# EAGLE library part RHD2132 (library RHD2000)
Intan Technologies RHD2132 chip
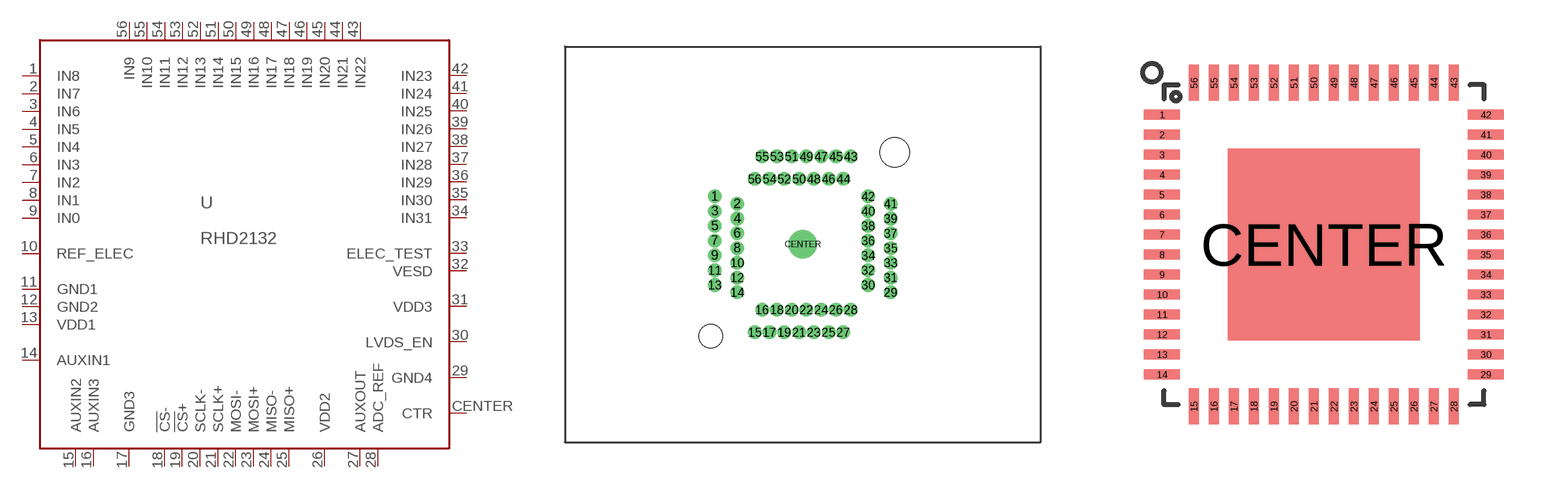
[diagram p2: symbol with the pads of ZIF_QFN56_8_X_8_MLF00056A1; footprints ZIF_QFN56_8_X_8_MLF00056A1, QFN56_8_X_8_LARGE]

Designator prefix U

## RHD2132_ZIF  [ZIF_QFN56_8_X_8_MLF00056A1]
1  IN8  in
2  IN7  in
3  IN6  in
4  IN5  in
5  IN4  in
6  IN3  in
7  IN2  in
8  IN1  in
9  IN0  in
10  REF_ELEC  in
11  GND1  pwr
12  GND2  pwr
13  VDD1  pwr
14  AUXIN1  in
15  AUXIN2  in
16  AUXIN3  in
17  GND3  pwr
18  !CS!-  in
19  !CS!+  in
20  SCLK-  in
21  SCLK+  in
22  MOSI-  in
23  MOSI+  in
24  MISO-  out
25  MISO+  out
26  VDD2  pwr
27  AUXOUT  hiz
28  ADC_REF  pas
29  GND4  pwr
30  LVDS_EN  in
31  VDD3  pwr
32  VESD  pwr
33  ELEC_TEST  in
34  IN31  in
35  IN30  in
36  IN29  in
37  IN28  in
38  IN27  in
39  IN26  in
40  IN25  in
41  IN24  in
42  IN23  in
43  IN22  in
44  IN21  in
45  IN20  in
46  IN19  in
47  IN18  in
48  IN17  in
49  IN16  in
50  IN15  in
51  IN14  in
52  IN13  in
53  IN12  in
54  IN11  in
55  IN10  in
56  IN9  in
CENTER  CTR  pwr

## RHD2132_QFN  [QFN56_8_X_8_LARGE]
Pads as for ZIF_QFN56_8_X_8_MLF00056A1

## RHD2132_COB  [RHD2000_56PIN_COB]
Pads as for ZIF_QFN56_8_X_8_MLF00056A1

## Footprint ZIF_QFN56_8_X_8_MLF00056A1 (pad centres in mm)
drill 0.41 pad 0.813: 1 -5.955,3.25; 2 -4.43,2.75; 3 -5.955,2.25; 4 -4.43,1.75; 5 -5.955,1.25; 6 -4.43,0.75; 7 -5.955,0.25; 8 -4.43,-0.25; 9 -5.955,-0.75; 10 -4.43,-1.25; 11 -5.955,-1.75; 12 -4.43,-2.25; 13 -5.955,-2.75; 14 -4.43,-3.25; 15 -3.25,-5.955; 16 -2.75,-4.43; 17 -2.25,-5.955; 18 -1.75,-4.43; 19 -1.25,-5.955; 20 -0.75,-4.43; 21 -0.25,-5.955; 22 0.25,-4.43; 23 0.75,-5.955; 24 1.25,-4.43; 25 1.75,-5.955; 26 2.25,-4.43; 27 2.75,-5.955; 28 3.25,-4.43; 29 5.955,-3.25; 30 4.43,-2.75; 31 5.955,-2.25; 32 4.43,-1.75; 33 5.955,-1.25; 34 4.43,-0.75; 35 5.955,-0.25; 36 4.43,0.25; 37 5.955,0.75; 38 4.43,1.25; 39 5.955,1.75; 40 4.43,2.25; 41 5.955,2.75; 42 4.43,3.25; 43 3.25,5.955; 44 2.75,4.43; 45 2.25,5.955; 46 1.75,4.43; 47 1.25,5.955; 48 0.75,4.43; 49 0.25,5.955; 50 -0.25,4.43; 51 -0.75,5.955; 52 -1.25,4.43; 53 -1.75,5.955; 54 -2.25,4.43; 55 -2.75,5.955; 56 -3.25,4.43
drill 1.2 pad 1.93: CENTER 0,0
hole 2 at 6.225,6.225
hole 1.6 at -6.225,-6.225

## Footprint QFN56_8_X_8_LARGE (pad centres in mm)
smd 0.9 x 0.25: 1 -4.05,3.25; 2 -4.05,2.75; 3 -4.05,2.25; 4 -4.05,1.75; 5 -4.05,1.25; 6 -4.05,0.75; 7 -4.05,0.25; 8 -4.05,-0.25; 9 -4.05,-0.75; 10 -4.05,-1.25; 11 -4.05,-1.75; 12 -4.05,-2.25; 13 -4.05,-2.75; 14 -4.05,-3.25; 29 4.05,-3.25; 30 4.05,-2.75; 31 4.05,-2.25; 32 4.05,-1.75; 33 4.05,-1.25; 34 4.05,-0.75; 35 4.05,-0.25; 36 4.05,0.25; 37 4.05,0.75; 38 4.05,1.25; 39 4.05,1.75; 40 4.05,2.25; 41 4.05,2.75; 42 4.05,3.25
smd 0.25 x 0.9: 15 -3.25,-4.05; 16 -2.75,-4.05; 17 -2.25,-4.05; 18 -1.75,-4.05; 19 -1.25,-4.05; 20 -0.75,-4.05; 21 -0.25,-4.05; 22 0.25,-4.05; 23 0.75,-4.05; 24 1.25,-4.05; 25 1.75,-4.05; 26 2.25,-4.05; 27 2.75,-4.05; 28 3.25,-4.05; 43 3.25,4.05; 44 2.75,4.05; 45 2.25,4.05; 46 1.75,4.05; 47 1.25,4.05; 48 0.75,4.05; 49 0.25,4.05; 50 -0.25,4.05; 51 -0.75,4.05; 52 -1.25,4.05; 53 -1.75,4.05; 54 -2.25,4.05; 55 -2.75,4.05; 56 -3.25,4.05
smd 4.8 x 4.8: CENTER 0,0

## Footprint RHD2000_56PIN_COB (pad centres in mm)
smd 0.203 x 0.152: 1 -3.048,2.134; 2 -3.048,1.829; 3 -3.048,1.524; 4 -3.048,1.219; 5 -3.048,0.914; 6 -3.048,0.61; 7 -3.048,0.305; 8 -3.048,0; 9 -3.048,-0.305; 10 -3.048,-0.61; 11 -3.048,-0.914; 12 -3.048,-1.524; 13 -3.048,-1.829; 14 -3.048,-2.134; 29 3.048,-2.134; 30 3.048,-1.829; 31 3.048,-1.524; 32 3.048,-0.914; 33 3.048,-0.61; 34 3.048,-0.305; 35 3.048,0; 36 3.048,0.305; 37 3.048,0.61; 38 3.048,0.914; 39 3.048,1.219; 40 3.048,1.524; 41 3.048,1.829; 42 3.048,2.134
smd 0.152 x 0.203: 15 -2.286,-2.692; 16 -1.981,-2.692; 17 -1.067,-2.692; 18 -0.762,-2.692; 19 -0.457,-2.692; 20 -0.152,-2.692; 21 0.152,-2.692; 22 0.457,-2.692; 23 0.762,-2.692; 24 1.067,-2.692; 25 1.372,-2.692; 26 1.676,-2.692; 27 1.981,-2.692; 28 2.286,-2.692; 43 2.286,2.692; 44 1.981,2.692; 45 1.676,2.692; 46 1.372,2.692; 47 1.067,2.692; 48 0.762,2.692; 49 0.457,2.692; 50 -0.457,2.692; 51 -0.762,2.692; 52 -1.067,2.692; 53 -1.372,2.692; 54 -1.676,2.692; 55 -1.981,2.692; 56 -2.286,2.692
smd 5.334 x 4.572: CENTER 0,0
